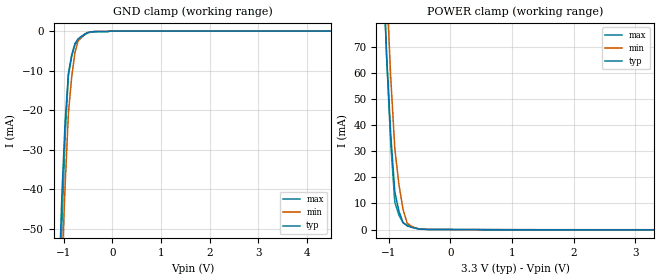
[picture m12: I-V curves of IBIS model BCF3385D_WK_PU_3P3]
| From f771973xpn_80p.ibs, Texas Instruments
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|BCF3385D_WK_PD_3P3; WEAK_PULLDOWN_ON
|   Model Cell BCF3385D_WK_PU_3P3
|BCF3385D_WK_PU_3P3
[Model]   BCF3385D_WK_PU_3P3
Model_type   Input
Polarity   Non-Inverting
Vinl =  0.8
Vinh =  2
C_comp   1.187844p   1.059102p   1.312744p
[Model Spec]
Vinl   0.8   0.8   0.8
Vinh   2   2   2
[Temperature Range]   25   155   -40
[Voltage Range]   3.3   2.97   3.63
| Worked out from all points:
|   GND clamp passes 1 mA (typ) near -0.60 V on its own axis
|   POWER clamp passes 1 mA (typ) near -0.65 V on its own axis
| Nom Voltages:
|   VDD=1.2, VDDS=3.3, VSS=0
| Min Voltages:
|   VDD=1.08, VDDS=2.97, VSS=0
| Max Voltages:
|   VDD=1.32, VDDS=3.63, VSS=0
[POWER_clamp]
|   voltage   I(typ)   I(min)   I(max)
-3.3V     1.862A     2.383A     2.005A
-1.1V     105.6mA    134.9mA    109.7mA
-1.033V   67.08mA    93.26mA    66.46mA
-966.7mV  36.7mA     58.63mA    33.38mA
-900mV    14.41mA    31.04mA    10.44mA
-833.3mV  7.024mA    17.26mA    5.478mA
-766.7mV  2.681mA    7.741mA    2.569mA
-700mV    1.383mA    2.484mA    1.712mA
-566.7mV  468.6uA    561.1uA    583.3uA
-366.7mV  39.94uA    41.02uA    52.49uA
3.3V      -108.8uA   -62.42uA   -174uA
[GND_clamp]
|   voltage   I(typ)   I(min)   I(max)
-3.3V     -1.421A    -1.358A    -2.122A
-1.1V     -65.93mA   -84.59mA   -78.36mA
-1.033V   -41.1mA    -60.01mA   -48.67mA
-966.7mV  -22.69mA   -38.72mA   -26.28mA
-900mV    -10.7mA    -20.74mA   -11.2mA
-833.3mV  -6.074mA   -11.65mA   -6.435mA
-766.7mV  -3.16mA    -5.542mA   -3.512mA
-700mV    -1.953mA   -2.407mA   -2.428mA
-566.7mV  -762.5uA   -790.2uA   -966.2uA
-500mV    -336.5uA   -374.5uA   -431.5uA
-33.33mV  0A         0A         0A
6.6V      0A         0A         0A
